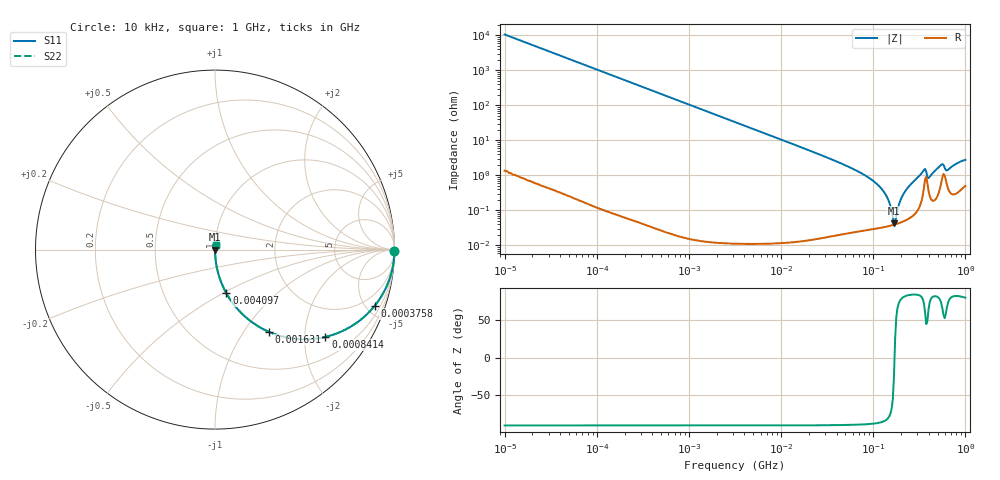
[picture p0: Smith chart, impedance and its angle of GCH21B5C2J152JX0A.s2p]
!Murata Part Number: GCH21B5C2J152JX0A
!These Parameters are Measured in Series Mode Connection
!Data Generated on Jun 19, 2026
!  o--ll--o
!Port1  Port2
!  o------o
!Operation Temp=25[degC], DC Bias Voltage=0[V]
!Freq. Start=10[kHz] Stop=1000[MHz] 401[Steps]
# Hz S RI R 50
!Freq.(Hz) S11(Real) S11(Imag) S21(Real) S21(Imag) S12(Real) S12(Imag) S22(Real) S22(Imag)
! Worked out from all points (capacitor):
!   401 points, 10 kHz to 1 GHz, reference 50 ohm
!   read as one part in series: C = 1.5 nF near 10.59 kHz
!   lowest |Z| = 43.1 mohm at 167.9 MHz (marker M1)
!   series resonance near 170.3 MHz, so ESL is about 580 pH
!   S11 on the Smith chart (normalised r, x): 10 kHz: open; 375.8 kHz: 1.00, -5.66; 841.4 kHz: 1.00, -2.53; 1.631 MHz: 1.00, -1.30; 4.097 MHz: 1.00, -0.52; 1 GHz: 1.01, +0.05
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10000  0.9999 -0.00941  8.97e-05 0.00941  8.97e-05 0.00941  0.9999 -0.00941
68786  0.9958 -0.0644  0.00418 0.0644  0.00418 0.0644  0.9958 -0.0644
375837  0.8889 -0.3142  0.1111 0.3142  0.1111 0.3142  0.8889 -0.3142
473151  0.8347 -0.3714  0.1653 0.3714  0.1653 0.3714  0.8347 -0.3714
841395  0.6149 -0.4865  0.3851 0.4865  0.3851 0.4865  0.6149 -0.4865
1631173  0.2982 -0.4574  0.7018 0.4574  0.7018 0.4574  0.2982 -0.4574
3162278  0.1016 -0.3019  0.8984 0.3019  0.8984 0.3019  0.1016 -0.3019
4097321  0.0631 -0.243  0.9369 0.243  0.9369 0.243  0.0631 -0.243
2.175204e7  0.00245 -0.0479  0.9976 0.0479  0.9976 0.0479  0.00245 -0.0479
8.912509e7  0.000352 -0.00866  0.9996 0.00866  0.9996 0.00866  0.000352 -0.00866
1.223207e8  0.000338 -0.00423  0.9997 0.00423  0.9997 0.00423  0.000338 -0.00423
1.372461e8  0.000349 -0.00274  0.9997 0.00274  0.9997 0.00274  0.000349 -0.00274
1.496236e8  0.000363 -0.00164  0.9996 0.00164  0.9996 0.00164  0.000363 -0.00164
1.678804e8  0.000391 -0.000181  0.9996 0.000181  0.9996 0.000181  0.000391 -0.000181
1.778279e8  0.000409 0.00055  0.9996 -0.00055  0.9996 -0.00055  0.000409 0.00055
1.938653e8  0.000445 0.00166  0.9996 -0.00166  0.9996 -0.00166  0.000445 0.00166
2.175204e8  0.000511 0.0032  0.9995 -0.0032  0.9995 -0.0032  0.000511 0.0032
3.447466e8  0.00287 0.0124  0.9971 -0.0124  0.9971 -0.0124  0.00287 0.0124
4.097321e8  0.00268 0.0087  0.9973 -0.0087  0.9973 -0.0087  0.00268 0.0087
5.463866e8  0.00633 0.019  0.9937 -0.019  0.9937 -0.019  0.00633 0.019
6.493816e8  0.00436 0.0138  0.9956 -0.0138  0.9956 -0.0138  0.00436 0.0138
1e9  0.00571 0.0272  0.9943 -0.0272  0.9943 -0.0272  0.00571 0.0272
